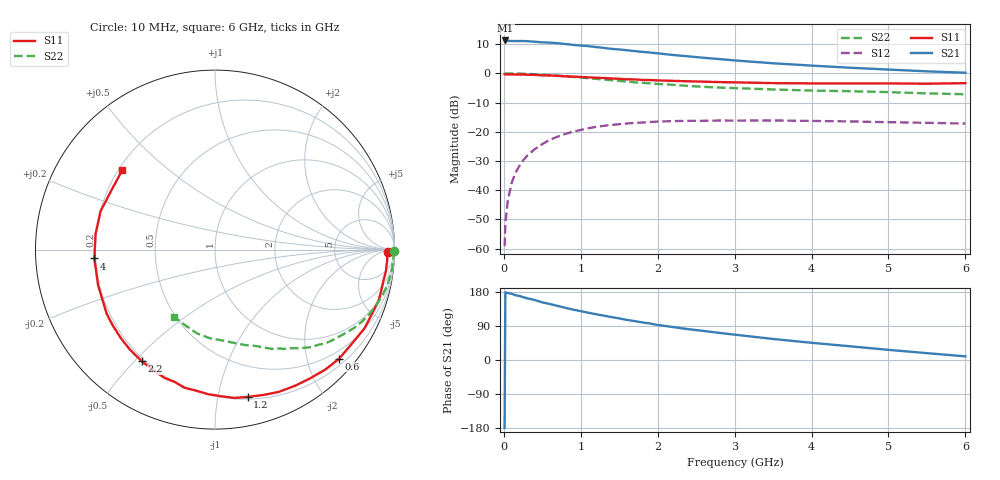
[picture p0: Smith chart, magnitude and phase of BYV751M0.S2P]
! SIEMENS Small Signal Semiconductors
! BFY420
! Si NPN RF SIEGET Grounded Emitter Transistor in MICRO-X
! VCE = 0.75 V  IC = 1 mA
! Common Emitter S-Parameters:  October  1996
# GHz  S  MA  R  50
!  f  S11  S21  S12  S22
! GHz  MAG  ANG  MAG  ANG  MAG  ANG  MAG  ANG
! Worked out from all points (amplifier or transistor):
!   36 points, 10 MHz to 6 GHz, reference 50 ohm
!   highest |S21| = 11.3 dB at 20 MHz (marker M1)
!   |S21| within 3 dB of that: start of sweep to 1.461 GHz
!   unconditionally stable (mu >= 1): 4.542 GHz to end of sweep
!   at 250 MHz: K = 0.05, MSG = 20.4 dB, |S12| = -29.8 dB
!   at 1.4 GHz: K = 0.24, MSG = 13.0 dB, |S12| = -17.7 dB
!   at 6 GHz: K = 1.33, MAG = 5.3 dB, |S12| = -17.2 dB
!   S11 on the Smith chart (normalised r, x): 10 MHz: 46, -17; 600 MHz: 0.33, -2.62; 1.2 GHz: 0.22, -1.22; 2.2 GHz: 0.19, -0.53; 4 GHz: 0.20, -0.04; 6 GHz: 0.22, +0.35
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0.01  0.9625 -0.8  3.649 -179.3  0.0011 86.2  0.9986 -0.4
0.02  0.9581 -1.6  3.66 178.6  0.0027 87.2  0.9959 -0.8
0.05  0.9612 -3.4  3.584 176.8  0.0064 89.9  0.9963 -1.9
0.1  0.9597 -7.2  3.586 174.9  0.0131 86.4  0.9933 -3.9
0.15  0.9542 -10.6  3.577 171.0  0.0197 82.8  0.992 -5.9
0.2  0.954 -14.1  3.573 169.0  0.0258 81.1  0.9903 -7.8
0.3  0.9473 -20.8  3.558 163.1  0.0384 76.7  0.9804 -11.7
0.5  0.9253 -34.6  3.399 152.1  0.0615 68.3  0.9503 -19.0
0.6  0.9207 -41.3  3.358 147.6  0.0731 64.1  0.9331 -22.6
0.8  0.8914 -53.8  3.182 137.7  0.0918 55.5  0.8902 -29.3
1.1  0.8538 -71.5  2.924 124.7  0.1149 45.3  0.8256 -37.8
1.2  0.8406 -77.5  2.819 120.7  0.1215 41.8  0.8047 -40.6
1.6  0.7923 -98.0  2.486 105.7  0.1387 30.8  0.723 -49.5
2  0.7578 -115.8  2.204 92.6  0.1495 21.7  0.6592 -56.7
2.2  0.7439 -123.2  2.063 86.9  0.1522 17.7  0.6364 -60.3
2.4  0.7315 -130.4  1.956 81.3  0.154 14.5  0.609 -63.6
2.8  0.7094 -143.4  1.758 71.6  0.1557 8.5  0.5712 -69.3
3.5  0.6809 -163.1  1.489 55.5  0.1562 0.6  0.5305 -78.5
4  0.6738 -175.8  1.359 45.4  0.1534 -4.0  0.507 -85.7
4.5  0.6712 172.7  1.249 36.2  0.1504 -8.2  0.4951 -93.1
5.5  0.6652 149.8  1.083 18.1  0.1424 -12.8  0.4542 -110.9
6  0.68 139.4  1.026 9.6  0.1382 -13.7  0.439 -121.1
